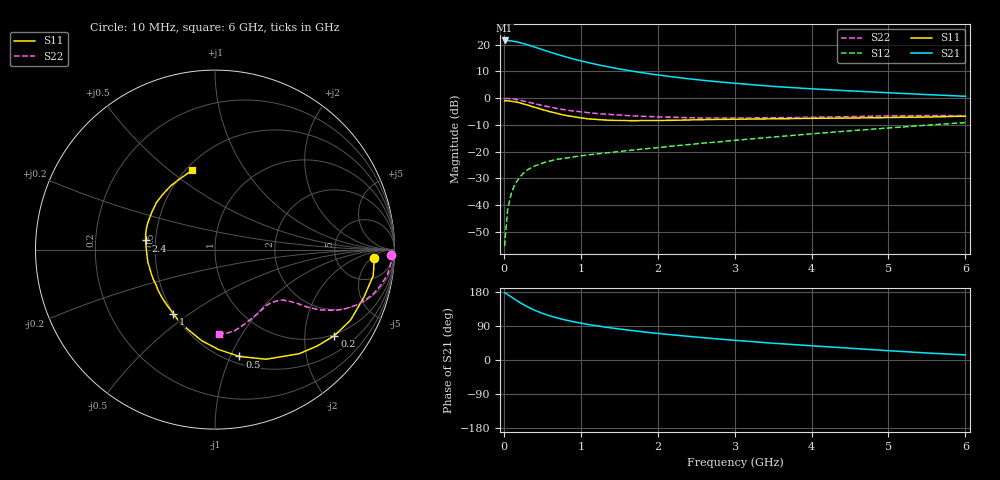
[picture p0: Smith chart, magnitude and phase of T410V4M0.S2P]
! Infineon Technologies  Discrete & RF Semiconductors
! BFR182T
! Si NPN RF Bipolar Junction Transistor in SC75
! VCE = 10 V  IC = 4 mA
! Common Emitter S-Parameters:  October  1999
# GHz  S  MA  R  50
!  f  S11  S21  S12  S22
! GHz  MAG  ANG  MAG  ANG  MAG  ANG  MAG  ANG
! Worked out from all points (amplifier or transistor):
!   36 points, 10 MHz to 6 GHz, reference 50 ohm
!   highest |S21| = 21.6 dB at 10 MHz (marker M1)
!   |S21| within 3 dB of that: start of sweep to 456.9 MHz
!   unconditionally stable (mu >= 1): 1.657 GHz to 4.277 GHz
!   at 250 MHz: K = 0.23, MSG = 24.3 dB, |S12| = -28.2 dB
!   at 1.4 GHz: K = 0.93, MSG = 15.9 dB, |S12| = -20.3 dB
!   at 6 GHz: K = 0.85, MSG = 4.9 dB, |S12| = -9.2 dB
!   S11 on the Smith chart (normalised r, x): 10 MHz: 14, -6; 200 MHz: 0.96, -2.80; 500 MHz: 0.57, -1.08; 1 GHz: 0.50, -0.43; 2.4 GHz: 0.44, +0.05; 6 GHz: 0.54, +0.60
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0.01  0.8844 -2.9  11.96 177.4  0.0017 82.4  0.9825 -1.6
0.02  0.8891 -2.4  11.86 177.1  0.0027 95.3  0.9795 -1.6
0.05  0.8935 -9.4  11.9 172.7  0.0083 87.9  0.9831 -4.1
0.1  0.8704 -18.0  11.69 166.1  0.0173 79.7  0.9715 -8.3
0.15  0.8513 -27.5  11.39 159.1  0.0253 74.9  0.9455 -12.0
0.2  0.82 -35.8  11.01 152.7  0.032 72.8  0.9182 -15.4
0.25  0.7829 -43.3  10.5 146.8  0.0388 67.8  0.8852 -18.4
0.3  0.7457 -51.1  10.01 141.2  0.0449 65.2  0.8532 -21.0
0.4  0.6733 -65.1  9.02 131.3  0.0537 59.1  0.7854 -25.2
0.5  0.6109 -77.1  8.076 123.3  0.0607 56.0  0.728 -27.7
0.6  0.5561 -88.2  7.24 116.4  0.0669 53.7  0.6785 -29.7
0.7  0.513 -98.2  6.538 110.7  0.0716 52.1  0.6361 -31.0
0.8  0.4748 -107.2  5.94 105.6  0.0753 50.6  0.6024 -32.0
1  0.4267 -123.0  4.966 97.5  0.0831 50.3  0.5542 -33.0
1.1  0.4087 -131.0  4.602 93.6  0.0868 50.3  0.5334 -33.8
1.5  0.3818 -154.6  3.514 81.8  0.1002 52.1  0.4828 -36.0
2.2  0.3844 178.1  2.49 66.2  0.1269 55.6  0.4377 -41.7
2.4  0.3898 172.5  2.299 62.4  0.135 56.4  0.4294 -43.8
3.5  0.4094 149.2  1.656 44.3  0.1867 58.5  0.4291 -56.5
4.5  0.4236 133.3  1.365 31.1  0.2441 57.3  0.4494 -69.8
5.5  0.4423 114.8  1.163 18.5  0.3114 53.9  0.4706 -82.0
6  0.4592 106.2  1.081 13.4  0.348 51.0  0.4701 -87.2
